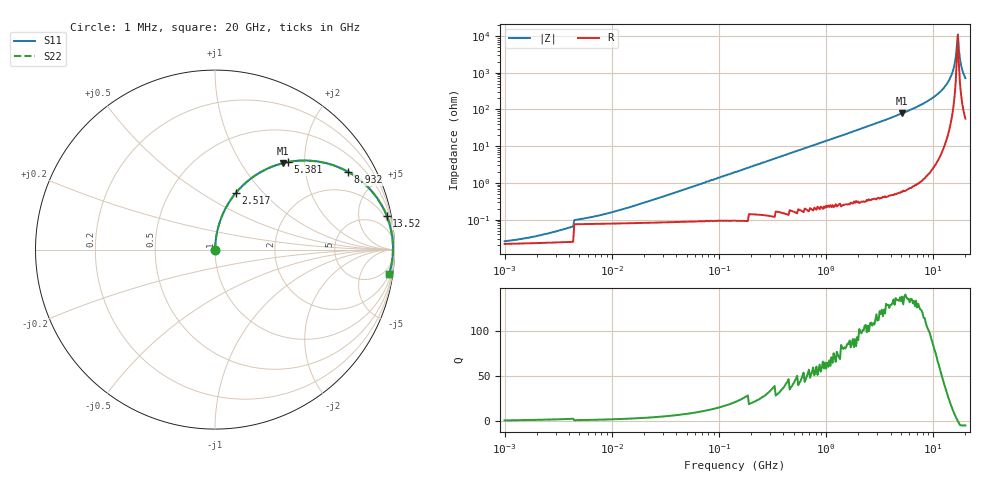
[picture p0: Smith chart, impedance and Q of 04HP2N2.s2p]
# MHz S MA R 50
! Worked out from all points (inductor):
!   431 points, 1 MHz to 20 GHz, reference 50 ohm
!   read as one part in series: L = 2.2 nH near 17.8 MHz
!   highest Q = 137 at 5.139 GHz (marker M1), where L = 2.42 nH
!   self-resonance near 16.63 GHz
!   S11 on the Smith chart (normalised r, x): 1 MHz: 1.00, +0.00; 2.517 GHz: 1.01, +0.71; 5.381 GHz: 1.01, +1.65; 8.932 GHz: 1.04, +3.41; 13.52 GHz: 1, +10; 20 GHz: 2, -14
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1  0.0004581 17.5  1 -0.0  1 -0.0  0.0004581 17.5
2.399  0.0005736 35.3  1 -0.0  1 -0.0  0.0005736 35.3
5.25  0.0008869 54.8  0.999 -0.0  0.999 -0.0  0.0008869 54.8
27.564  0.003868 79.7  0.999 -0.2  0.999 -0.2  0.003868 79.7
144.716  0.02 85.8  0.999 -1.1  0.999 -1.1  0.02 85.8
742.485  0.102 83.1  0.993 -5.9  0.993 -5.9  0.102 83.1
2516.601  0.334 69.9  0.939 -19.5  0.939 -19.5  0.334 69.9
3898.162  0.493 60.0  0.866 -29.5  0.866 -29.5  0.493 60.0
5139.119  0.614 51.7  0.785 -37.9  0.785 -37.9  0.614 51.7
5381.378  0.635 50.2  0.768 -39.4  0.768 -39.4  0.635 50.2
8931.947  0.859 30.2  0.503 -59.2  0.503 -59.2  0.859 30.2
11245.28  0.936 19.7  0.338 -69.4  0.338 -69.4  0.936 19.7
13520.39  0.975 11.0  0.191 -77.1  0.191 -77.1  0.975 11.0
15170.55  0.988 5.4  0.095 -80.1  0.095 -80.1  0.988 5.4
15885.69  0.991 3.2  0.056 -78.8  0.056 -78.8  0.991 3.2
16255.8  0.991 2.1  0.037 -75.4  0.037 -75.4  0.991 2.1
16634.54  0.992 1.0  0.019 -62.7  0.019 -62.7  0.992 1.0
17022.1  0.991 -0.2  0.008994 17.1  0.008994 17.1  0.991 -0.2
17418.69  0.991 -1.3  0.024 66.9  0.024 66.9  0.991 -1.3
17824.53  0.99 -2.4  0.043 75.2  0.043 75.2  0.99 -2.4
18664.78  0.987 -4.6  0.081 78.4  0.081 78.4  0.987 -4.6
20000  0.98 -7.9  0.138 77.5  0.138 77.5  0.98 -7.9
